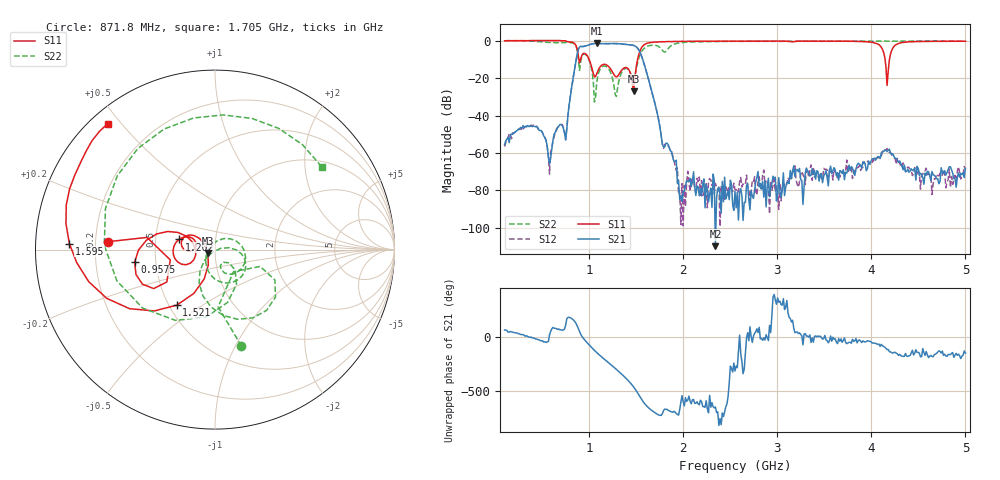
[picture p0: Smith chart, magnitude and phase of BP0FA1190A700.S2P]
! s2p File.  Ports: 1,3
# MHz S DB R 50
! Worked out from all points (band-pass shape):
!   401 points, 100 MHz to 5 GHz, reference 50 ohm
!   highest |S21| = -1.45 dB at 1.08 GHz (marker M1); lowest = -109.9 dB at 2.342 GHz (marker M2)
!   |S21| within 3 dB of the highest: 885.7 MHz to 1.521 GHz (635.6 MHz wide, 52.8 % of centre)
!   lowest |S11| = -27.1 dB at 1.472 GHz (marker M3), VSWR 1.09, Z = 46.1 - j1.7 ohm
!   |S11| at or under -10 dB: 889.9 MHz to 907.3 MHz (17.44 MHz wide, 1.94 % of centre); 998.5 MHz to 1.514 GHz (515.9 MHz wide, 41.1 % of centre); 4.146 GHz to 4.192 GHz (46.82 MHz wide, 1.12 % of centre)
!   |S22| runs from -32.8 to 0.0 dB; largest |S21 - S12| = 0.0027
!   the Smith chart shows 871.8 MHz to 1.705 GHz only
!   S11 on the Smith chart (normalised r, x): 871.8 MHz: 0.25, +0.03; 957.5 MHz: 0.38, -0.07; 1.202 GHz: 0.66, +0.08; 1.521 GHz: 0.55, -0.39; 1.595 GHz: 0.10, +0.02; 1.705 GHz: 0.05, +0.46
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100  -0.03 -10.4  -55.50 69.0  -56.59 66.4  -0.03 -32.4
320.5  0.05 -34.6  -45.82 10.7  -45.80 20.8  -0.07 -112.5
590  0.13 -74.1  -62.59 56.3  -59.50 71.1  -0.98 115.6
773.75  -0.52 -120.5  -39.88 -174.7  -39.83 -172.9  -0.82 14.1
871.75  -4.48 175.8  -7.13 107.7  -7.12 107.8  -5.07 -74.7
920.75  -7.86 -147.6  -3.06 11.5  -3.06 11.5  -8.54 -26.9
957.5  -6.88 -171.1  -2.85 -30.1  -2.86 -30.1  -7.23 -60.9
1080  -17.65 -154.2  -1.45 -141.5  -1.45 -141.6  -22.11 7.8
1202.5  -13.60 164.3  -1.54 126.8  -1.54 126.9  -14.80 -80.8
1361.75  -14.87 176.7  -1.82 4.4  -1.81 4.4  -15.67 -2.9
1472  -27.12 -155.3  -2.51 -100.8  -2.51 -100.8  -21.54 -57.0
1521  -8.49 -124.6  -4.43 -165.5  -4.42 -165.5  -10.38 -76.6
1594.5  -1.81 177.6  -14.24 98.5  -14.24 98.5  -3.72 159.4
1704.75  -0.71 130.4  -34.82 16.0  -34.78 16.2  -2.47 37.8
1741.5  -0.62 121.3  -43.40 -2.7  -43.09 -2.3  -3.23 -4.7
1839.5  -0.43 100.6  -55.58 41.4  -56.17 48.6  -4.22 150.0
1986.5  -0.31 79.5  -85.97 178.4  -76.43 104.7  -0.97 47.0
2341.75  -0.25 48.8  -109.86 73.2  -76.35 75.4  -0.39 -15.9
2550  -0.18 37.1  -80.56 47.7  -79.50 -170.1  -0.32 -36.6
3370.75  -0.16 6.1  -68.32 -5.6  -74.69 19.7  -0.22 -96.6
4191.5  -10.23 48.5  -57.96 -131.7  -59.81 -125.9  -0.21 -139.9
5000  -0.28 -32.5  -68.35 -146.1  -68.87 -145.6  -0.11 -163.7
